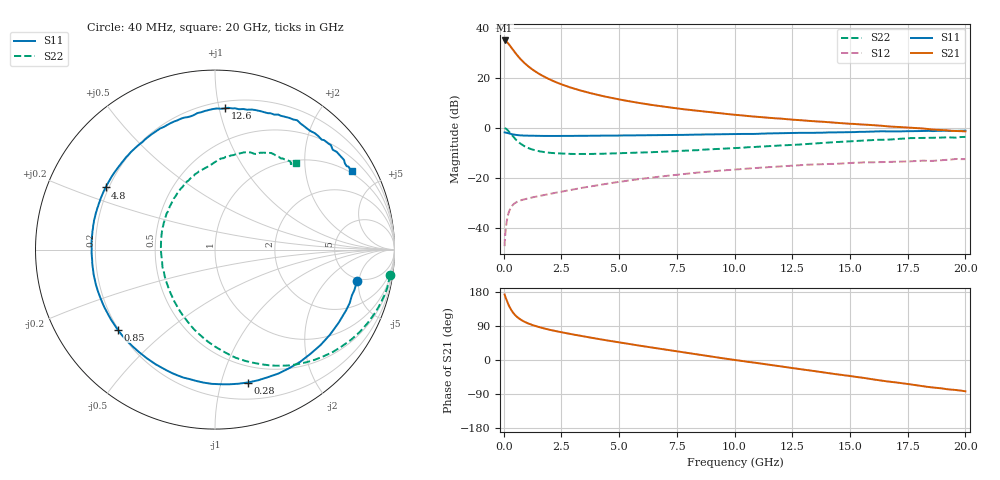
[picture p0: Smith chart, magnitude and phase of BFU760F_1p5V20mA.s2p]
! Filename:  P:\Prog\Test\Noise\ATS_data\Testdata_Net\Split files Spar\BFU760F_2W_C1_Bias5_1.5V_5mA_60mA_D.s2p
! Date/Time: Mon 06/Feb/2012 15:07:28
! BFU760_2W_C1_Bias5_1.5V_5mA_60mA_R.s2p
! MDIF S-parameter v. bias file
! BFU760_2W_C1_1.5V_5mA_60mA
! Date/time Fri Mar 18 11:09:37 2011
! VAR V_out= 1.5002
! VAR I_out= 20.0400
! VAR V_in= 0.7911
! VAR I_in= 0.0625
! Device data file deembeded for feedlines and parallel
! Original file: \Split files Spar\BFU760_2W_C1_Bias5_1.5V_5mA_60mA_R.s2p
! Feed-files: PR003V01_101208_Feed1.s2p, PR003V01_101208_Feed2.s2p
! Parallel-file: PR003V01_101208_Par.s2p
# MHz S MA R 50
!  Freq-MHz  S11-mag  S11-arg  S21-mag  S21-arg  S12-mag  S12-arg  S22-mag  S22-arg
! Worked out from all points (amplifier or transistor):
!   167 points, 40 MHz to 20 GHz, reference 50 ohm
!   highest |S21| = 34.9 dB at 40 MHz (marker M1)
!   |S21| within 3 dB of that: start of sweep to 345.2 MHz
!   unconditionally stable (mu >= 1): 4.321 GHz to 14.07 GHz; 14.25 GHz to 14.83 GHz
!   at 550 MHz: K = 0.24, MSG = 29.5 dB, |S12| = -29.7 dB
!   at 4.2 GHz: K = 0.99, MSG = 17.8 dB, |S12| = -22.7 dB
!   at 20 GHz: K = 0.91, MSG = 5.5 dB, |S12| = -12.5 dB
!   S11 on the Smith chart (normalised r, x): 40 MHz: 4.61, -4.73; 280 MHz: 0.34, -1.21; 850 MHz: 0.20, -0.35; 4.8 GHz: 0.19, +0.26; 12.6 GHz: 0.25, +1.04; 20 GHz: 0.93, +3.53
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40  0.811 -12.5  55.29 172.9  0.004354 84.2  0.9873 -8.3
50  0.8085 -16.3  55.07 170.5  0.005901 82.7  0.9835 -10.7
90  0.8019 -27.8  53.77 163.8  0.00961 77.0  0.966 -19.3
160  0.7875 -47.5  50.03 152.7  0.01602 67.7  0.9093 -33.5
220  0.7758 -62.9  46.73 144.4  0.02051 61.1  0.8486 -44.4
280  0.7624 -76.3  43 137.1  0.02411 55.5  0.7881 -54.0
400  0.7391 -98.1  36.23 125.5  0.02906 47.3  0.6738 -70.1
500  0.7251 -111.7  31.42 118.3  0.03177 42.6  0.6 -81.0
650  0.7108 -126.6  25.82 110.2  0.03451 38.3  0.5157 -94.2
850  0.7017 -140.6  20.62 102.5  0.03703 35.3  0.4434 -107.9
1050  0.6955 -150.3  17.06 96.8  0.0391 34.2  0.3978 -118.8
1250  0.6928 -157.7  14.51 92.2  0.041 33.9  0.3682 -127.7
1800  0.6889 -171.7  10.22 82.5  0.04615 34.6  0.3256 -146.1
2500  0.6894 176.6  7.362 73.3  0.0532 36.2  0.3079 -162.2
3400  0.6929 165.2  5.438 63.0  0.06358 36.4  0.3013 -176.7
4800  0.701 150.4  3.843 48.5  0.08101 34.1  0.3086 165.6
6800  0.7152 132.3  2.699 29.3  0.1067 26.9  0.3322 145.2
10200  0.7537 104.6  1.787 -1.5  0.1495 9.0  0.4004 115.6
12600  0.7889 85.9  1.444 -22.1  0.1771 -5.4  0.4579 96.8
13400  0.7933 80.3  1.357 -28.7  0.1855 -11.2  0.4829 90.9
16800  0.8482 54.4  1.055 -57.7  0.2097 -32.7  0.5854 65.8
20000  0.8775 29.8  0.851 -82.6  0.2371 -54.1  0.6589 46.8
